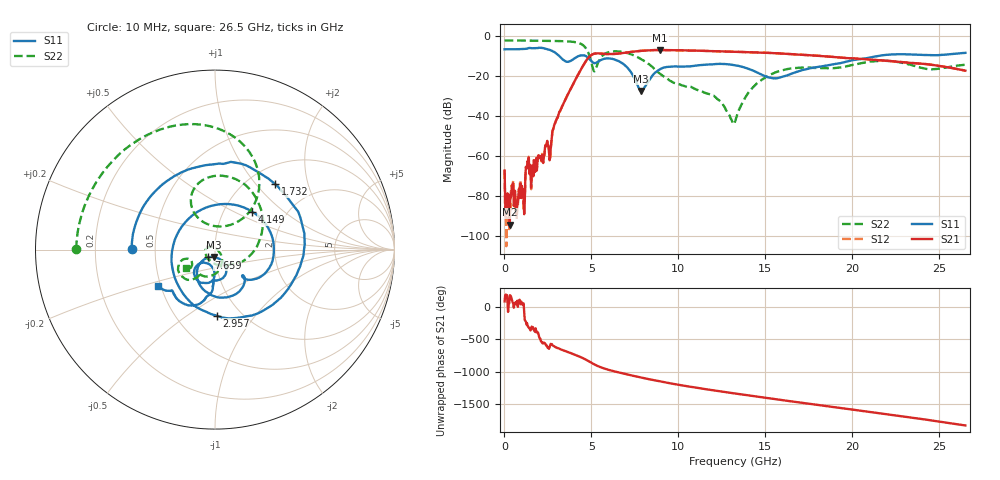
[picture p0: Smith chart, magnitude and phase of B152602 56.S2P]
!  2-Port S-parameters saved by WinCal
! VAR MeasName=S-Parameters (CALIBRATED_DATA) read from VNA (N5242A)
! VAR MeasDate=2016-1-5 16:33:56
! VAR NAME=B152602 56
! VAR FILENAME=B152602 56.S2P
! VAR DATE=2016-1-5 16:33:56
! VAR PHYS_PORTS=1,2
# Hz S DB R 50
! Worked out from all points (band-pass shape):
!   801 points, 10 MHz to 26.5 GHz, reference 50 ohm
!   highest |S21| = -7.02 dB at 8.95 GHz (marker M1); lowest = -94.6 dB at 308 MHz (marker M2)
!   |S21| within 3 dB of the highest: 4.926 GHz to 18.21 GHz (13.29 GHz wide, 115 % of centre)
!   lowest |S11| = -27.6 dB at 7.858 GHz (marker M3), VSWR 1.09, Z = 49.1 - j4.06 ohm
!   |S11| at or under -10 dB: 3.146 GHz to 4.278 GHz (1.132 GHz wide, 30.5 % of centre); 4.666 GHz to 21.48 GHz (16.81 GHz wide, 129 % of centre)
!   |S22| runs from -44.1 to -2.2 dB; largest |S21 - S12| = 0.0035
!   S11 on the Smith chart (normalised r, x): 10 MHz: 0.37, +0.01; 1.732 GHz: 1.31, +1.27; 2.957 GHz: 0.77, -0.66; 4.149 GHz: 1.36, +0.63; 7.659 GHz: 0.92, -0.08; 26.5 GHz: 0.48, -0.23
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1e7  -6.67 179.3  -67.44 84.0  -67.22 124.5  -2.24 179.8
3.080125e8  -6.66 157.5  -94.61 177.3  -90.19 -36.0  -2.25 175.2
1.036488e9  -6.55 103.9  -79.00 53.6  -77.00 59.0  -2.30 164.0
1.367612e9  -6.08 79.7  -63.88 54.9  -63.80 54.6  -2.33 158.7
1.73185e9  -6.11 47.4  -64.81 -13.9  -64.45 -10.9  -2.36 152.8
2.625888e9  -7.04 -43.8  -61.04 124.4  -60.88 127.0  -2.45 136.7
2.957012e9  -8.68 -88.5  -42.56 95.2  -42.62 95.3  -2.51 129.7
3.4537e9  -12.43 -178.6  -32.71 42.6  -32.72 42.4  -2.63 117.6
4.149062e9  -10.58 45.5  -20.78 -28.0  -20.78 -27.9  -3.22 93.1
4.447075e9  -9.69 4.9  -16.00 -62.3  -15.99 -62.3  -4.19 76.9
5.17555e9  -13.60 -43.7  -8.85 -168.0  -8.84 -168.0  -17.72 87.3
6.202038e9  -11.44 -85.6  -9.07 93.4  -9.06 93.5  -7.76 91.3
7.658988e9  -24.78 -130.6  -7.59 1.8  -7.58 1.8  -10.63 25.3
7.857662e9  -27.55 -100.1  -7.44 -10.0  -7.44 -9.9  -11.58 15.3
8.851038e9  -17.19 -63.0  -7.03 -65.0  -7.01 -65.0  -18.32 -42.9
8.950375e9  -16.63 -65.9  -7.02 -70.2  -7.01 -70.2  -18.97 -49.7
1.103646e10  -14.80 -98.1  -7.35 -166.8  -7.34 -166.6  -26.89 169.6
1.3255e10  -14.69 -128.0  -7.93 105.0  -7.91 104.8  -43.05 31.4
1.471195e10  -19.04 -136.9  -8.31 49.5  -8.28 49.5  -22.44 -58.6
1.769208e10  -15.98 -92.0  -9.73 -60.4  -9.70 -60.2  -15.93 -121.3
2.209604e10  -9.32 -114.4  -12.53 141.7  -12.45 141.6  -12.51 -149.0
2.65e10  -8.45 -147.6  -17.38 -28.0  -17.37 -28.3  -14.40 -147.4
